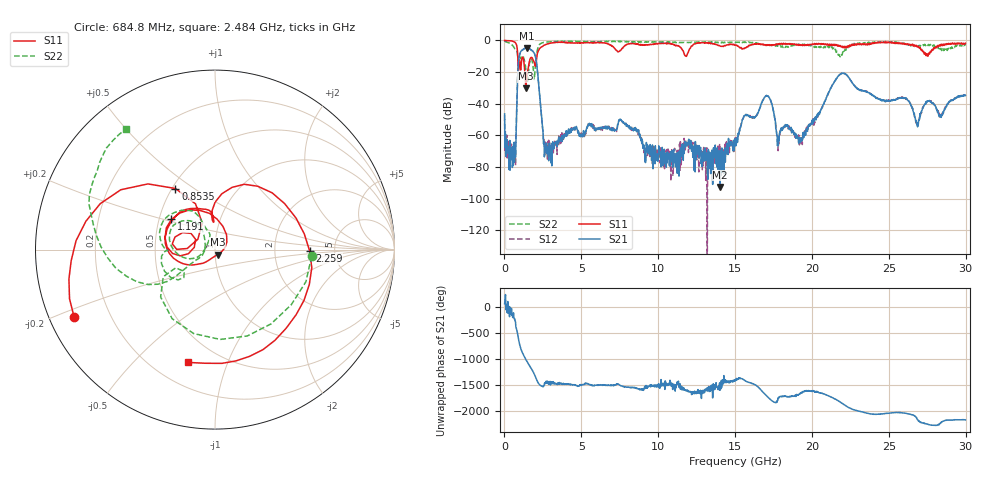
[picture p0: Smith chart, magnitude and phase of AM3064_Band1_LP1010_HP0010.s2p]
# Hz S DB R 50.0
!freq dBS11 angS11 dBS21 angS21 dBS12 angS12 dBS22 angS22
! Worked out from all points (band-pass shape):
!   1600 points, 10 MHz to 29.98 GHz, reference 50 ohm
!   highest |S21| = -4.76 dB at 1.453 GHz (marker M1); lowest = -92.6 dB at 14.03 GHz (marker M2)
!   |S21| within 3 dB of the highest: 1.028 GHz to 1.924 GHz (895.4 MHz wide, 60.7 % of centre)
!   lowest |S11| = -30.2 dB at 1.397 GHz (marker M3), VSWR 1.06, Z = 51.3 - j2.84 ohm
!   |S11| at or under -10 dB: 865.7 MHz to 2.111 GHz (1.245 GHz wide, 83.7 % of centre); 11.80303 GHz to 11.84017 GHz (37.14 MHz wide, 0.314 % of centre)
!   |S22| runs from -25.9 to -0.4 dB; largest |S21 - S12| = 0.0073
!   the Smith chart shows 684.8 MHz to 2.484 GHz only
!   S11 on the Smith chart (normalised r, x): 684.8 MHz: 0.07, -0.22; 853.5 MHz: 0.52, +0.42; 1.191 GHz: 0.58, +0.21; 2.259 GHz: 3.23, -0.06; 2.484 GHz: 0.34, -0.73
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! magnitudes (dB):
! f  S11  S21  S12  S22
! 10 MHz  0.0  -46.4  -47.3  -0.4
! 441.1 MHz  -0.3  -72.9  -66.2  -2.4
! 684.8 MHz  -1.2  -68.5  -72.1  -5.3
! 853.5 MHz  -7.8  -24.7  -24.7  -9.7
! 1.191 GHz  -10.6  -6.0  -5.9  -9.6
! 1.397 GHz  -30.2  -4.8  -4.8  -18.6
! 1.453 GHz  -21.2  -4.8  -4.7  -21.3
! 2.259 GHz  -5.6  -31.3  -31.3  -2.9
! 2.484 GHz  -3.8  -55.7  -56.0  -1.6
! 2.934 GHz  -1.8  -65.0  -63.8  -0.9
! 5.015 GHz  -1.4  -60.1  -61.2  -0.7
! 7.582 GHz  -6.0  -50.0  -50.3  -0.6
! 10 GHz  -2.0  -73.1  -73.6  -1.0
! 14.03 GHz  -3.6  -92.6  -68.9  -1.3
! 15 GHz  -2.9  -64.8  -60.6  -1.3
! 17.03 GHz  -3.0  -34.9  -35.0  -3.2
! 17.82 GHz  -2.3  -66.2  -66.0  -3.4
! 19.99 GHz  -2.7  -51.4  -52.4  -3.2
! 21.94 GHz  -4.1  -20.8  -20.9  -9.4
! 25 GHz  -1.1  -38.1  -38.4  -1.1
! 26.83 GHz  -4.0  -53.1  -52.5  -3.4
! 29.98 GHz  -1.8  -34.7  -34.6  -3.2
